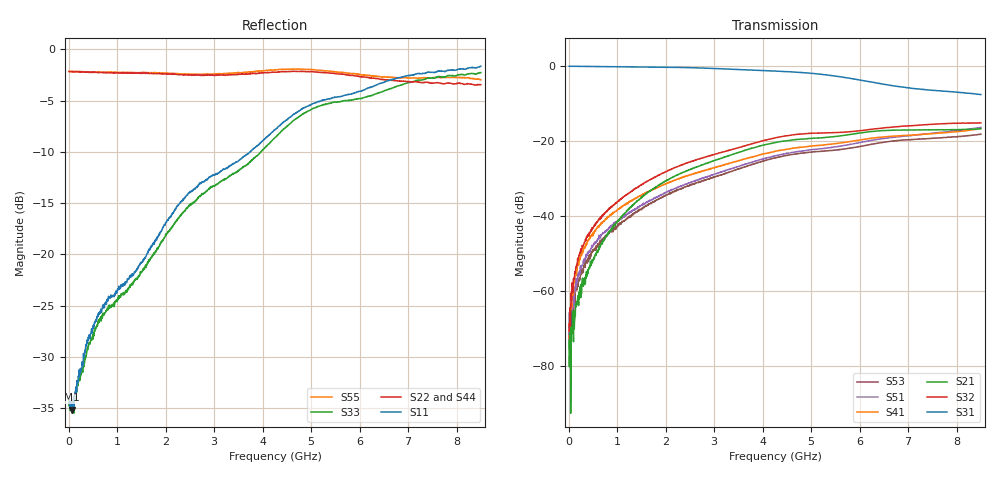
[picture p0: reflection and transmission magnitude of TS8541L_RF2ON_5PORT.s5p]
! Created with skrf (http://scikit-rf.org).
# Hz S RI R 50.0
!freq ReS11 ImS11 ReS12 ImS12 ReS13 ImS13
! ReS14 ImS14 ReS15 ImS15
! ReS21 ImS21 ReS22 ImS22 ReS23 ImS23
! ReS24 ImS24 ReS25 ImS25
! ReS31 ImS31 ReS32 ImS32 ReS33 ImS33
! ReS34 ImS34 ReS35 ImS35
! ReS41 ImS41 ReS42 ImS42 ReS43 ImS43
! ReS44 ImS44 ReS45 ImS45
! ReS51 ImS51 ReS52 ImS52 ReS53 ImS53
! ReS54 ImS54 ReS55 ImS55
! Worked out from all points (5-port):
!   1601 points, 10 MHz to 8.5 GHz, reference 50 ohm
!   strongest paths, dB at 10 MHz, 2.132 GHz, 4.255 GHz, 6.378 GHz, 8.5 GHz:
!     S31: -0.1, -0.4, -1.4, -4.7, -7.7
!     S32: -70.7, -27.4, -19.2, -16.7, -15.2
!     S21: -73.1, -29.8, -20.5, -17.3, -16.8
!     S41: -71.9, -30.7, -22.8, -19.1, -16.7
!     S51: -75.3, -32.9, -24.0, -19.6, -16.4
!     S53: -74.9, -33.8, -24.5, -20.6, -18.2
!   lowest |S11| = -35.1 dB at 73.67 MHz (marker M1), VSWR 1.04, Z = 51.7 - j0.56 ohm
!   |S11| at or under -10 dB: start of sweep to 3.743 GHz
